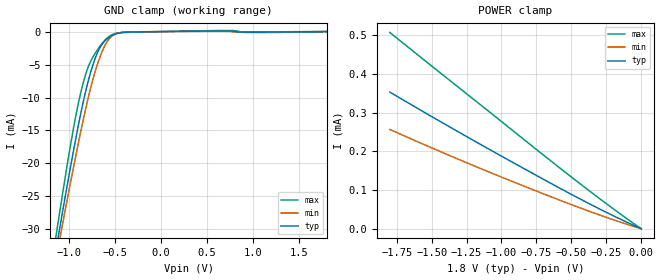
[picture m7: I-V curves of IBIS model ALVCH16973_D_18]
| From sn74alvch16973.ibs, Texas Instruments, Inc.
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[Model]   ALVCH16973_D_18
Model_type  Input
Vinl=0.5775
Vinh=1.2675
| variable   typ   min   max
C_comp   2.43pF   2.00pF   2.86pF
[Temperature Range]   40   100   -40
| Ambient temperature   25   85   -40
[Voltage range]   1.8   1.65   1.95
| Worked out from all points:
|   GND clamp passes 1 mA (typ) near -0.57 V on its own axis
[GND Clamp]
| ALVCH16973_D_18
|   Voltage   I(typ)   I(min)   I(max)
-1.8V     -90.83mA   -87.48mA   -94.81mA
-1.145V   -33.72mA   -35.09mA   -31.65mA
-1.125V   -32.08mA   -33.57mA   -29.83mA
-1.09V    -29.22mA   -30.93mA   -26.68mA
-1.06V    -26.79mA   -28.69mA   -24.02mA
-935mV    -17.09mA   -19.64mA   -13.66mA
-830mV    -9.883mA   -12.6mA    -7.138mA
-770mV    -6.559mA   -8.991mA   -4.746mA
-690mV    -3.26mA    -5.018mA   -2.8mA
-545mV    -717.7uA   -844.4uA   -595uA
-355mV    -81.09uA   -57.95uA   -118.9uA
1.8V      135.5pA    17.04uA    -35.19uA
[POWER Clamp]
| ALVCH16973_D_18
|   Voltage   I(typ)   I(min)   I(max)
-1.8V     353.2uA    256.5uA    507.2uA
-1.225V   233uA      166.7uA    341.5uA
-645mV    116.8uA    82.3uA     174.6uA
-280mV    47.69uA    33.08uA    72.78uA
-16.28fV  135.5pA    810.7pA    36.51pA
